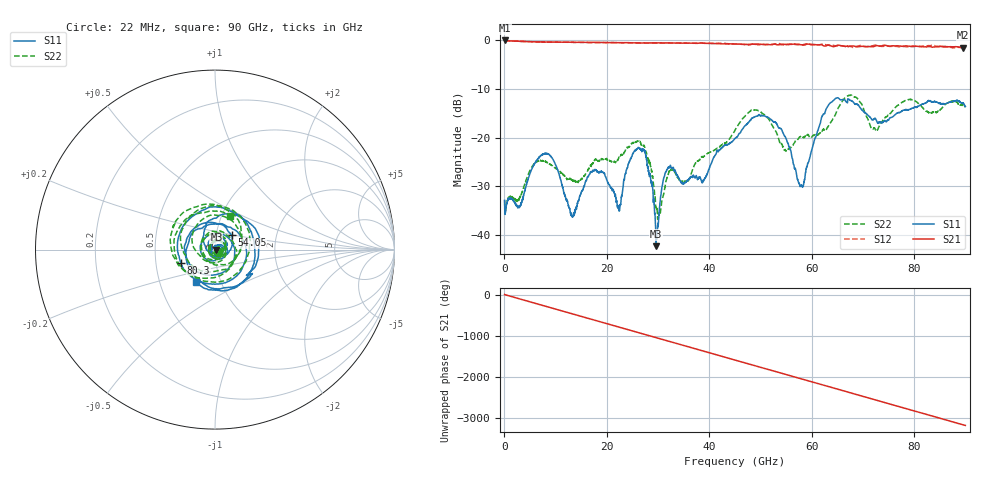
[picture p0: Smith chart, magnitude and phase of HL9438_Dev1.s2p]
! 4/1/2022 11:05:40 AM
! C:\USERS\VECTORSTARUSER\DESKTOP\JASON\100GDCB\AS21.S2P
! CHANNEL.1
! TR.MEASUREMENT
! CORRECTED.DATA
! RF.CORRECTION: FULL.TWO.PORT.CAL.PORT.1.2
! AVERAGING.OFF
! IF.BANDWIDTH: 1KHZ
! SWEEPTYPE:  FREQ.SWEEP(Linear)
! Reference Plane Port Info
! PORT:  PORT1  PORT2
! DISTANCE:  0  m  0  m
! TIME:  0  s  0  s
! PHASE.OFFSET:  0 °  0 °
! LOSS:  0  dB  0  dB
! REF.LOSS:  0  dB  0  dB
! REF.FREQ:  0  Hz  0  Hz
! Power Info
! POWER:  -10  dBm  -10  dBm
! EFF.POWER:  -10  dBm  -10  dBm
! POWER(>54G):  -10  dBm  -10  dBm
! EFF.POWER(>54G):  -10  dBm  -10  dBm
! SOURCE.ATTEN:  0  dB  0  dB
! TEST.ATTEN:  0  dB  0  dB
# GHZ S RI R 50.0
! FREQ.GHZ  S11RE  S11IM  S21RE  S21IM  S12RE  S12IM  S22RE  S22IM
!; PortSelection: Port_12
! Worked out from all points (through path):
!   4091 points, 22 MHz to 90 GHz, reference 50 ohm
!   highest |S21| = -0.14 dB at 66 MHz (marker M1); lowest = -1.6 dB at 89.52 GHz (marker M2)
!   group delay of S21, straight-line fit = 98.3 ps
!   lowest |S11| = -42.2 dB at 29.59 GHz (marker M3), VSWR 1.02, Z = 50.8 + j0.0198 ohm
!   |S11| at or under -10 dB: start of sweep to end of sweep
!   |S22| runs from -36.7 to -11.3 dB; largest |S21 - S12| = 0.041
!   S11 on the Smith chart (normalised r, x): 22 MHz: 1.03, -0.03; 54.05 GHz: 1.19, +0.19; 80.3 GHz: 0.67, -0.10; 90 GHz: 0.76, -0.29
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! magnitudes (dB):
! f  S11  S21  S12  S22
! 22 MHz  -32.8  -0.2  -0.2  -32.8
! 66 MHz  -35.5  -0.1  -0.1  -35.6
! 7.876 GHz  -23.3  -0.5  -0.5  -24.8
! 13.22 GHz  -36.0  -0.5  -0.5  -28.8
! 15.03 GHz  -31.1  -0.5  -0.5  -28.4
! 19.12 GHz  -27.1  -0.6  -0.6  -24.4
! 22.35 GHz  -34.9  -0.6  -0.6  -24.0
! 26.86 GHz  -22.7  -0.7  -0.6  -21.5
! 29.59 GHz  -42.2  -0.6  -0.6  -34.3
! 30.03 GHz  -37.8  -0.6  -0.6  -35.4
! 32.01 GHz  -26.1  -0.6  -0.7  -27.4
! 38.83 GHz  -29.0  -0.7  -0.7  -23.9
! 45.01 GHz  -20.2  -0.9  -0.9  -18.5
! 49.48 GHz  -15.6  -0.9  -1.0  -14.5
! 54.05 GHz  -18.3  -0.9  -1.0  -21.2
! 57.88 GHz  -29.8  -1.0  -1.0  -19.7
! 60.02 GHz  -22.5  -1.0  -1.0  -19.9
! 64.79 GHz  -11.9  -1.2  -1.3  -14.9
! 75.02 GHz  -16.4  -1.3  -1.3  -15.6
! 80.3 GHz  -13.8  -1.3  -1.3  -12.6
! 89.52 GHz  -13.0  -1.6  -1.5  -13.3
! 90 GHz  -13.7  -1.5  -1.4  -13.8
